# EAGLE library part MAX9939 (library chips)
spi programmable differential amplifier
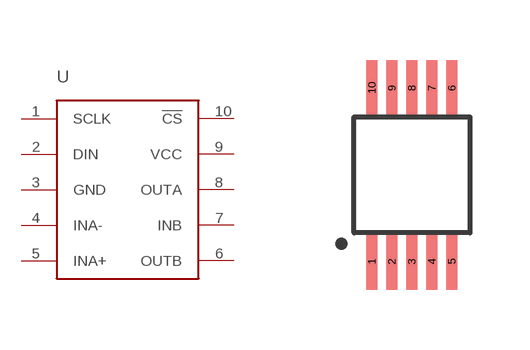
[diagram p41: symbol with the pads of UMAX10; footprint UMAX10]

Designator prefix -

## MAX9939 (DIGIKEY: MAX9939AUB+-ND)  [UMAX10]
1  SCLK
2  DIN
3  GND
4  INA-
5  INA+
6  OUTB
7  INB
8  OUTA
9  VCC
10  !CS

## Footprint UMAX10 (pad centres in mm)
smd 0.28 x 1.4: 1 -1,-2.17; 2 -0.5,-2.17; 3 0,-2.17; 4 0.5,-2.17; 5 1,-2.17; 6 1,2.17; 7 0.5,2.17; 8 0,2.17; 9 -0.5,2.17; 10 -1,2.17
